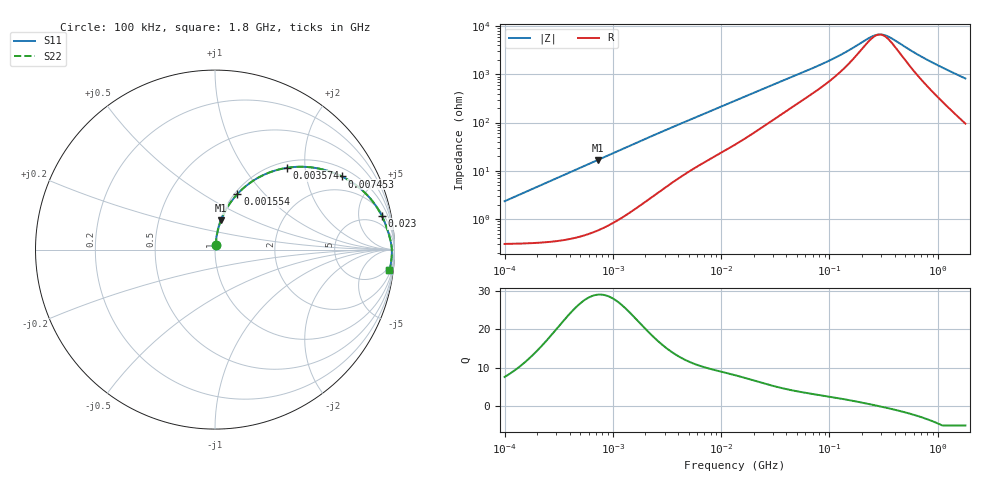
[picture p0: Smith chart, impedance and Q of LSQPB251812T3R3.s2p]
! LSQPB251812T3R3  S-PARAMETER MODEL  ( General Type )
! Model Generated by TAIYO YUDEN Corporation (http://www.ty-top.com)
! Version 3.0
! TAIYO YUDEN Control No. 110926NF18SB-HKC
! Copyright(c) 2007 TAIYO YUDEN CO.,LTD. All Rights Reserved.
! Product Description (link to TY-COMPAS)
! https://ds.yuden.co.jp/TYCOMPAS/or/detail?pn=LSQPB251812T3R3M&u=M
! Products Name : Inductors
! Characteristics :
!  Inductance : 3.3 uH , SRF(min) : 70 MHz , DC Resistance(max) : 0.39 Ohm
!  Rated Current : Saturation :800 mA , Temp Rise : 580 mA (40 degC)
!  Case Size : 2.5 x 1.8 / 0.098 x 0.071 [mm/inch] , Thickness : 1.2 / 0.048 [mm/inch]
!  (Conditions: Temperature = 25 degC , DC Bias Current/Voltage = 0A / 0V)
! External Node Assignments :
!  1  o---GGG---o  2
! GND o---------o GND
! Frequency Range : 0.1MHz  -  1800MHz  [ 402 STEP ]
# MHz S RI R 50
! Freq[MHz].  S11 Real  S11 Imag  S21 Real  S21 Imag  S12 Real  S12 Imag  S22 Real  S22 Imag
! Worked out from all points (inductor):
!   401 points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, 100 kHz to 1.8 GHz, reference 50 ohm
!   read as one part in series: L = 3.7 uH near 105 kHz
!   highest Q = 29 at 727.3 kHz (marker M1), where L = 3.69 uH
!   self-resonance near 289.1 MHz
!   S11 on the Smith chart (normalised r, x): 100 kHz: 1.01, +0.05; 1.554 MHz: 1.03, +0.72; 3.574 MHz: 1.12, +1.61; 7.453 MHz: 1.33, +3.23; 23 MHz: 2.50, +9.33; 1.8 GHz: 3, -16
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0.1  0.00358 0.0231  0.9964 -0.0231  0.9964 -0.0231  0.00358 0.0231
0.247521  0.00658 0.057  0.9934 -0.057  0.9934 -0.057  0.00658 0.057
0.516129  0.0184 0.1172  0.9816 -0.1172  0.9816 -0.1172  0.0184 0.1172
0.727265  0.033 0.1623  0.967 -0.1623  0.967 -0.1623  0.033 0.1623
1.102914  0.0689 0.2357  0.9311 -0.2357  0.9311 -0.2357  0.0689 0.2357
1.55409  0.1245 0.3094  0.8755 -0.3094  0.8755 -0.3094  0.1245 0.3094
2.034681  0.1918 0.3694  0.8082 -0.3694  0.8082 -0.3694  0.1918 0.3694
2.66389  0.2823 0.4212  0.7177 -0.4212  0.7177 -0.4212  0.2823 0.4212
3.574164  0.4026 0.4558  0.5974 -0.4558  0.5974 -0.4558  0.4026 0.4558
5.03627  0.5528 0.456  0.4472 -0.456  0.4472 -0.456  0.5528 0.456
7.452807  0.7065 0.4078  0.2935 -0.4078  0.2935 -0.4078  0.7065 0.4078
9.999495  0.796 0.3511  0.204 -0.3511  0.204 -0.3511  0.796 0.3511
13.41641  0.8613 0.2893  0.1387 -0.2893  0.1387 -0.2893  0.8613 0.2893
22.99727  0.9295 0.1878  0.0705 -0.1878  0.0705 -0.1878  0.9295 0.1878
38.46609  0.958 0.1189  0.042 -0.1189  0.042 -0.1189  0.958 0.1189
69.24595  0.9733 0.0684  0.0267 -0.0684  0.0267 -0.0684  0.9733 0.0684
124.6553  0.9812 0.0349  0.0188 -0.0349  0.0188 -0.0349  0.9812 0.0349
253.6402  0.985 0.00502  0.015 -0.00502  0.015 -0.00502  0.985 0.00502
301.0823  0.9853 -0.00157  0.0147 0.00157  0.0147 0.00157  0.9853 -0.00157
357.3983  0.9855 -0.00824  0.0145 0.00824  0.0145 0.00824  0.9855 -0.00824
782.6622  0.9839 -0.0453  0.0161 0.0453  0.0161 0.0453  0.9839 -0.0453
1800  0.9722 -0.1161  0.0278 0.1161  0.0278 0.1161  0.9722 -0.1161
